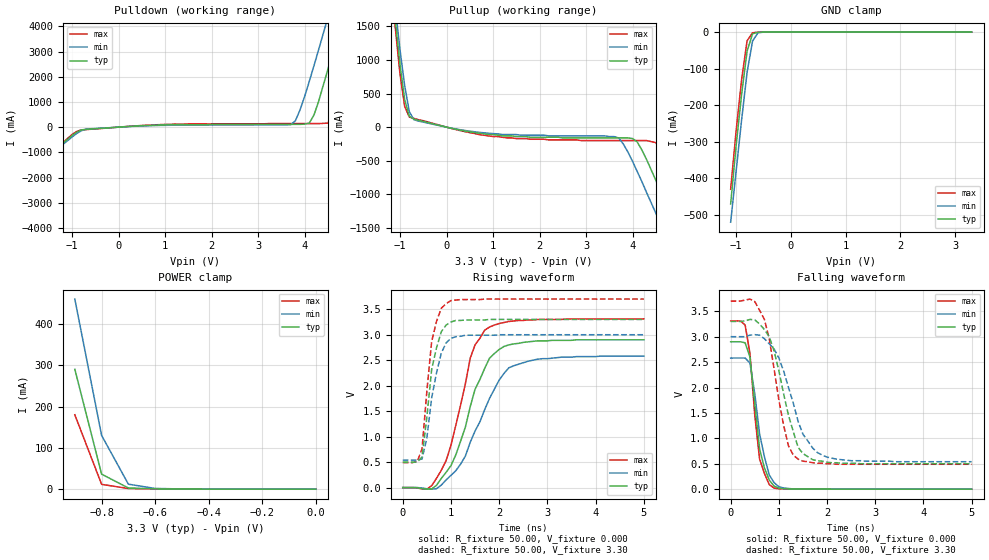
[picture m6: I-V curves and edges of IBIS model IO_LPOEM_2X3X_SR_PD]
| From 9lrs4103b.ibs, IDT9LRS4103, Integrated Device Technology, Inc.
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|   Model IO_LPOEM_2X3X_SR_PD
[Model]   IO_LPOEM_2X3X_SR_PD
Model_type   I/O
Polarity   Inverting
Enable   Active-High
Vinl =   0.35V
Vinh =   0.70V
Vmeas =   1.50V
Cref =  30.00pF
Rref =  0.000
Vref =   1.50V
C_comp   3.40pF   2.85pF   3.95pF
[Temperature Range]   27.00   70.00   0.000
[Voltage Range]   3.30V   3.00V   3.70V
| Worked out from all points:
|   slope of the pulldown table from 0 to 0.495 V, typ, clamps not added: 8.92 ohm
|   slope of the pullup table from 0 to 0.495 V, typ, clamps not added: 7.13 ohm
|   GND clamp passes 1 mA (typ) near -0.61 V on its own axis
|   POWER clamp passes 1 mA (typ) near -0.61 V on its own axis
|   rising waveform, R_fixture 50.00, V_fixture 0.000: 20-80 % time 619ps typ, 739ps min, 498ps max; typ from 0 V to 2.9 V
|   rising waveform, R_fixture 50.00, V_fixture 3.30: 20-80 % time 241ps typ, 258ps min, 215ps max; typ from 0.5 V to 3.3 V
|   falling waveform, R_fixture 50.00, V_fixture 0.000: 20-80 % time 226ps typ, 265ps min, 190ps max; typ from 2.9 V to 0 V
|   falling waveform, R_fixture 50.00, V_fixture 3.30: 20-80 % time 430ps typ, 509ps min, 355ps max; typ from 3.3 V to 0.5 V
[Pulldown]
| voltage   I(typ)   I(min)   I(max)
-3.3V     -4.16A     -4.01A     -4.26A
-3.1V     -3.82A     -3.69A     -3.9A
-800mV    -110mA     -140mA     -110mA
3.7V      110mA      100mA      140mA
3.9V      110mA      680mA      140mA
4.1V      160mA      1.82A      140mA
4.2V      480mA      2.44A      140mA
4.5V      2.3A       4.36A      160mA
4.7V      3.65A      5.67A      900mA
5.1V      6.43A      8.33A      3.62A
5.3V      7.83A      9.66A      5.05A
6.6V      17.08A     18.42A     14.59A
[Pullup]
| voltage   I(typ)   I(min)   I(max)
-3.3V     16.9A      16.26A     17.32A
-1.5V     4.22A      4.28A      4.19A
-1V       930mA      1.15A      790mA
-900mV    410mA      620mA      310mA
-700mV    120mA      110mA      130mA
1V        -110mA     -96.16mA   -140mA
3.7V      -160mA     -160mA     -200mA
4.1V      -220mA     -660mA     -200mA
4.5V      -790mA     -1.28A     -230mA
4.9V      -1.45A     -1.91A     -800mA
5.3V      -2.12A     -2.55A     -1.48A
6.6V      -4.33A     -4.64A     -3.76A
[GND_clamp]
| voltage   I(typ)   I(min)   I(max)
 | -3.30   -4.15A   -4.00A   -4.25A
  |-3.20   -3.98A   -3.84A   -4.07A
  |-3.10   -3.81A   -3.68A   -3.90A
  |-3.00   -3.64A   -3.52A   -3.72A
  |-2.90   -3.47A   -3.36A   -3.55A
  |-2.80   -3.30A   -3.20A   -3.37A
  |-2.70   -3.13A   -3.04A   -3.19A
  |-2.60   -2.96A   -2.88A   -3.02A
  |-2.50   -2.79A   -2.72A   -2.84A
  |-2.40   -2.62A   -2.56A   -2.67A
  |-2.30   -2.45A   -2.40A   -2.49A
  |-2.20   -2.29A   -2.24A   -2.32A
  |-2.10   -2.12A   -2.08A   -2.14A
  |-2.00   -1.95A   -1.92A   -1.97A
  |-1.90   -1.78A   -1.76A   -1.79A
  |-1.80   -1.61A   -1.61A   -1.62A
  |-1.70   -1.45A   -1.45A   -1.45A
  |-1.60   -1.28A   -1.29A   -1.27A
  |-1.50   -1.12A   -1.14A   -1.10A
  |-1.40   -0.95A   -0.98A   -0.93A
  |-1.30   -0.79A   -0.83A   -0.76A
  |-1.20   -0.63A   -0.67A   -0.59A
-1.1V     -470mA     -520mA     -430mA
-1V       -310mA     -380mA     -270mA
-900mV    -170mA     -240mA     -130mA
-800mV    -52.1mA    -110mA     -23.59mA
-700mV    -4.69mA    -24.29mA   -1.84mA
-600mV    -430uA     -1.9mA     -210uA
-400mV    -1.76uA    -10.19uA   -470nA
3.3V      150pA      24.14uA    -330pA
[POWER_clamp]
| voltage   I(typ)   I(min)   I(max)
  |-3.30   13.34A   12.83A   13.67A
  |-3.20   12.78A   12.30A   13.09A
  |-3.10   12.22A   11.77A   12.51A
  |-3.00   11.66A   11.24A   11.93A
  |-2.90   11.10A   10.71A   11.35A
  |-2.80   10.54A   10.18A   10.77A
  |-2.70   9.98A   9.66A   10.19A
  |-2.60   9.42A   9.13A   9.61A
  |-2.50   8.86A   8.60A   9.03A
  |-2.40   8.31A   8.07A   8.46A
  |-2.30   7.75A   7.54A   7.88A
  |-2.20   7.19A   7.02A   7.30A
  |-2.10   6.64A   6.49A   6.73A
  |-2.00   6.08A   5.97A   6.15A
  |-1.90   5.53A   5.45A   5.58A
  |-1.80   4.97A   4.92A   5.00A
  |-1.70   4.42A   4.40A   4.43A
  |-1.60   3.88A   3.89A   3.86A
  |-1.50   3.33A   3.37A   3.30A
  |-1.40   2.79A   2.86A   2.74A
  |-1.30   2.25A   2.35A   2.18A
  |-1.20   1.72A   1.85A   1.63A
  |-1.10   1.21A   1.37A   1.10A
  |-1.00   0.72A   0.90A   0.60A
-900mV    290mA      460mA      180mA
-800mV    36.29mA    130mA      11.65mA
-700mV    2.83mA     12.05mA    1.52mA
-600mV    760uA      1.75mA     430uA
-500mV    190uA      510uA      90.12uA
-400mV    36.78uA    130uA      14.36uA
-300mV    5.51uA     24.14uA    1.75uA
-200mV    600nA      3.69uA     140nA
-100mV    40.72nA    380nA      6.97nA
0V        150pA      200pA      160pA
[Ramp]
| variable   typ   min   max
dV/dt_r   1.74/0.61n   1.55/0.73n   1.99/0.50n
dV/dt_f   1.68/0.43n   1.47/0.52n   1.93/0.35n
R_load = 50.00
[Rising Waveform]
R_fixture = 50.00
V_fixture = 0.000
V_fixture_min = 0.000
V_fixture_max = 0.000
| time   V(typ)   V(min)   V(max)
0s        0V         1.58uV     0V
500ps     -31.08mV   -23.86mV   -31.47mV
800ps     180mV      48.86mV    340mV
900ps     300mV      150mV      530mV
1.1ns     640mV      330mV      1.22V
1.4ns     1.59V      890mV      2.54V
1.7ns     2.34V      1.53V      3.09V
2ns       2.71V      2.11V      3.22V
2.3ns     2.82V      2.39V      3.27V
5ns       2.9V       2.58V      3.31V
[Rising Waveform]
R_fixture = 50.00
V_fixture = 3.30
V_fixture_min = 3.00
V_fixture_max = 3.70
| time   V(typ)   V(min)   V(max)
0s        500mV      540mV      490mV
300ps     500mV      540mV      510mV
400ps     600mV      560mV      760mV
500ps     1.38V      970mV      1.89V
600ps     2.32V      1.76V      2.87V
700ps     2.74V      2.25V      3.26V
800ps     3.06V      2.64V      3.52V
900ps     3.19V      2.84V      3.61V
1.3ns     3.29V      2.99V      3.69V
5ns       3.3V       3V         3.7V
[Falling Waveform]
R_fixture = 50.00
V_fixture = 0.000
V_fixture_min = 0.000
V_fixture_max = 0.000
| time   V(typ)   V(min)   V(max)
0s        2.9V       2.58V      3.31V
300ps     2.88V      2.58V      3.23V
400ps     2.6V       2.48V      2.67V
500ps     1.68V      1.88V      1.46V
600ps     790mV      1.09V      590mV
700ps     420mV      640mV      310mV
800ps     180mV      280mV      90.94mV
900ps     60.16mV    130mV      21.56mV
1.3ns     3.67mV     4.29mV     2.65mV
5ns       -820nV     6.39uV     -990nV
[Falling Waveform]
R_fixture = 50.00
V_fixture = 3.30
V_fixture_min = 3.00
V_fixture_max = 3.70
| time   V(typ)   V(min)   V(max)
0s        3.3V       3V         3.7V
500ps     3.33V      3.04V      3.69V
700ps     3.14V      2.96V      3.34V
900ps     2.72V      2.76V      2.37V
1ns       2.33V      2.58V      1.75V
1.2ns     1.45V      2V         850mV
1.4ns     820mV      1.33V      590mV
1.7ns     580mV      810mV      520mV
2ns       530mV      630mV      500mV
5ns       500mV      540mV      490mV
